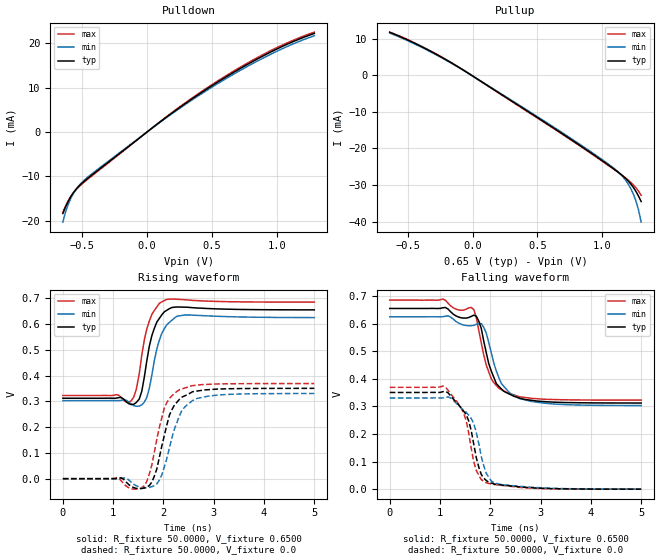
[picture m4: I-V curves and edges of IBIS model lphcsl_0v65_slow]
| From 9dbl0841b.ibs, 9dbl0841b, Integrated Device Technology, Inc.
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|   Model lphcsl_0v65_slow
[Model]  lphcsl_0v65_slow
Model_type Output
Polarity   Non-Inverting
Vmeas =  0.4000V
Cref =   2.0000pF
Rref =   0.0
Vref =   0.4000V
C_comp   1.1000pF   1.0000pF   1.2000pF
[Temperature Range]   27.0000   70.0000   0.0
[Voltage Range]   0.6500V   0.6200V   0.6800V
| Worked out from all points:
|   slope of the pulldown table from 0 to 0.098 V, typ, clamps not added: 44.2 ohm
|   slope of the pullup table from 0 to 0.098 V, typ, clamps not added: 43.9 ohm
|   rising waveform, R_fixture 50.0000, V_fixture 0.6500: 20-80 % time 217ps typ, 227ps min, 213ps max; typ from 0.312 V to 0.655 V
|   rising waveform, R_fixture 50.0000, V_fixture 0.0: 20-80 % time 300ps typ, 317ps min, 278ps max; typ from 0 V to 0.35 V
|   falling waveform, R_fixture 50.0000, V_fixture 0.6500: 20-80 % time 317ps typ, 367ps min, 305ps max; typ from 0.655 V to 0.312 V
|   falling waveform, R_fixture 50.0000, V_fixture 0.0: 20-80 % time 310ps typ, 318ps min, 297ps max; typ from 0.35 V to 0 V
[Pulldown]
|Voltage   I(typ)   I(min)   I(max)
-650mV    -18.4mA    -20.35mA   -18.11mA
-630mV    -16.96mA   -18.14mA   -16.75mA
-610mV    -15.72mA   -16.43mA   -15.59mA
-590mV    -14.65mA   -15.06mA   -14.6mA
-550mV    -12.99mA   -13.03mA   -13.08mA
-510mV    -11.76mA   -11.6mA    -11.93mA
-410mV    -9.338mA   -9.072mA   -9.537mA
50mV      1.142mA    1.099mA    1.173mA
370mV     7.923mA    7.656mA    8.116mA
690mV     13.82mA    13.41mA    14.11mA
990mV     18.55mA    18.04mA    18.87mA
1.29V     22.21mA    21.69mA    22.52mA
[Pullup]
|Voltage   I(typ)   I(min)   I(max)
-640mV    11.75mA    11.55mA    11.82mA
-380mV    7.586mA    7.409mA    7.685mA
-120mV    2.462mA    2.392mA    2.508mA
640mV     -14.77mA   -14.51mA   -14.93mA
1.06V     -24.87mA   -24.62mA   -24.99mA
1.16V     -27.56mA   -27.79mA   -27.55mA
1.2V      -28.91mA   -29.73mA   -28.67mA
1.22V     -29.72mA   -30.99mA   -29.29mA
1.24V     -30.67mA   -32.51mA   -29.98mA
1.26V     -31.78mA   -34.42mA   -30.78mA
1.28V     -33.06mA   -36.87mA   -31.72mA
1.3V      -34.52mA   -40.17mA   -32.83mA
[Ramp]
| variable   typ   min   max
dV/dt_r  0.2102/0.2996n   0.1982/0.3170n   0.2213/0.2779n
dV/dt_f  0.2056/0.3168n   0.1929/0.3668n   0.2173/0.3054n
R_load = 50.0000
[Rising Waveform]
R_fixture= 50.0000
V_fixture= 0.6500
V_fixture_min= 0.6200
V_fixture_max= 0.6800
|time   V(typ)   V(min)   V(max)
0s        312mV      302.7mV    322.6mV
1.16ns    315.1mV    303.7mV    314mV
1.36ns    287.6mV    289.2mV    302.4mV
1.46ns    295.2mV    280.7mV    346.1mV
1.57ns    339.5mV    286.4mV    480mV
1.72ns    514.4mV    351.1mV    611.8mV
1.87ns    607.8mV    504.4mV    666.5mV
2.07ns    653.5mV    597.6mV    695.4mV
2.42ns    665.2mV    634.9mV    694.1mV
5ns       654.7mV    624.7mV    684.7mV
[Rising Waveform]
R_fixture= 50.0000
V_fixture= 0.0
V_fixture_min= 0.0
V_fixture_max= 0.0
|time   V(typ)   V(min)   V(max)
0s        795.8nV    0V         1.025uV
1.16ns    3.353mV    966.2uV    -8.131mV
1.57ns    -38.26mV   -34.39mV   -35.46mV
1.72ns    -26.52mV   -33.6mV    18.59mV
1.92ns    83.62mV    -5.323mV   199.9mV
2.12ns    247mV      120mV      311mV
2.32ns    308mV      244.6mV    345.1mV
2.58ns    337.3mV    302.9mV    360.8mV
2.93ns    345.6mV    321.3mV    366.3mV
5ns       350.3mV    330.3mV    368.9mV
[Falling Waveform]
R_fixture= 50.0000
V_fixture= 0.6500
V_fixture_min= 0.6200
V_fixture_max= 0.6800
|time   V(typ)   V(min)   V(max)
0s        654.6mV    624.4mV    684.7mV
1.16ns    652.2mV    627.7mV    673.8mV
1.62ns    625.7mV    592.1mV    658.3mV
1.77ns    609.1mV    599.7mV    576mV
1.92ns    494mV      565.2mV    449.3mV
2.02ns    427.5mV    494.1mV    399.5mV
2.22ns    363mV      382.4mV    360.7mV
2.37ns    345.5mV    351.6mV    346.3mV
3.08ns    317.2mV    311.3mV    325.7mV
5ns       312mV      302.9mV    322.6mV
[Falling Waveform]
R_fixture= 50.0000
V_fixture= 0.0
V_fixture_min= 0.0
V_fixture_max= 0.0
|time   V(typ)   V(min)   V(max)
0s        350.3mV    330.4mV    368.9mV
1.11ns    354.3mV    332.9mV    368.9mV
1.46ns    284.9mV    287.4mV    278.9mV
1.52ns    270.1mV    278.3mV    249.4mV
1.62ns    212.7mV    256.1mV    149.6mV
1.77ns    80.26mV    166mV      50.77mV
1.92ns    31.43mV    57.65mV    23.38mV
2.07ns    19.39mV    24.27mV    17.15mV
2.37ns    12.4mV     13.79mV    10.82mV
5ns       28.57uV    81.91uV    11.78uV
